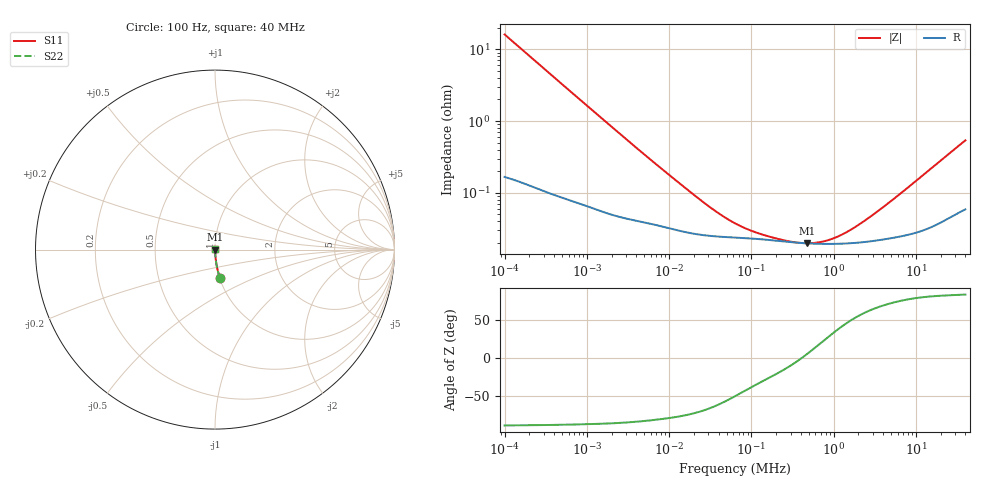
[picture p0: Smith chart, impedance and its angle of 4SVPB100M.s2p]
! Touchstone file from project
# GHZ S RI R 50.000000
! Modal data exported
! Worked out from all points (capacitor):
!   450 points, 100 Hz to 40 MHz, reference 50 ohm
!   read as one part in series: C = 98.8 uF near 105.9 Hz
!   lowest |Z| = 19.8 mohm at 473.2 kHz (marker M1)
!   series resonance near 412.2 kHz, so ESL is about 1.5 nH
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1e-07  0.0268 -0.1563  0.9732 0.1563  0.9732 0.1563  0.0268 -0.1563
1.059254e-07  0.0241 -0.148  0.9759 0.148  0.9759 0.148  0.0241 -0.148
1.584893e-07  0.0116 -0.1005  0.9884 0.1005  0.9884 0.1005  0.0116 -0.1005
2.511886e-07  0.00526 -0.064  0.9947 0.064  0.9947 0.064  0.00526 -0.064
4.340103e-07  0.0023 -0.0373  0.9977 0.0373  0.9977 0.0373  0.0023 -0.0373
8.659643e-07  0.00105 -0.0189  0.999 0.0189  0.999 0.0189  0.00105 -0.0189
7.498942e-06  0.000353 -0.0023  0.9996 0.0023  0.9996 0.0023  0.000353 -0.0023
2.985383e-05  0.000253 -0.000607  0.9997 0.000607  0.9997 0.000607  0.000253 -0.000607
4.466836e-05  0.000243 -0.000409  0.9998 0.000409  0.9998 0.000409  0.000243 -0.000409
6.493816e-05  0.000237 -0.000284  0.9998 0.000284  0.9998 0.000284  0.000237 -0.000284
0.0001  0.000231 -0.000185  0.9998 0.000185  0.9998 0.000185  0.000231 -0.000185
0.0001727826  0.000219 -0.000103  0.9998 0.000103  0.9998 0.000103  0.000219 -0.000103
0.0003072557  0.000205 -3.45e-05  0.9998 3.45e-05  0.9998 3.45e-05  0.000205 -3.45e-05
0.0004731513  0.000198 1.69e-05  0.9998 -1.69e-05  0.9998 -1.69e-05  0.000198 1.69e-05
0.0005463865  0.000196 3.53e-05  0.9998 -3.53e-05  0.9998 -3.53e-05  0.000196 3.53e-05
0.0006878599  0.000194 6.7e-05  0.9998 -6.7e-05  0.9998 -6.7e-05  0.000194 6.7e-05
0.0008413951  0.000194 9.79e-05  0.9998 -9.79e-05  0.9998 -9.79e-05  0.000194 9.79e-05
0.001059254  0.000194 0.000138  0.9998 -0.000138  0.9998 -0.000138  0.000194 0.000138
0.001333521  0.000196 0.000186  0.9998 -0.000186  0.9998 -0.000186  0.000196 0.000186
0.002304093  0.000205 0.00034  0.9998 -0.00034  0.9998 -0.00034  0.000205 0.00034
0.004731513  0.000231 0.000695  0.9998 -0.000695  0.9998 -0.000695  0.000231 0.000695
0.04  0.000616 0.00535  0.9994 -0.00535  0.9994 -0.00535  0.000616 0.00535
